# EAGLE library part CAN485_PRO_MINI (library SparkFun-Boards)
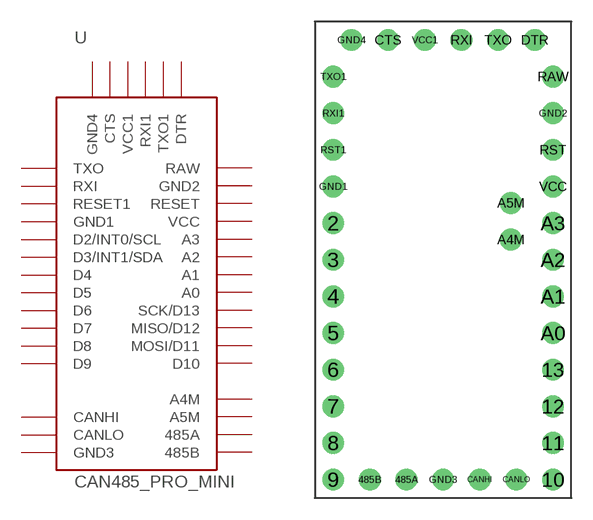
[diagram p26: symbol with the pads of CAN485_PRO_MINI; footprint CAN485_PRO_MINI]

Designator prefix -

## CAN485_PRO_MINIPRO_MINI_COMPATIBLE  [CAN485_PRO_MINI]
2  D2/INT0/SCL
3  D3/INT1/SDA
4  D4
5  D5
6  D6
7  D7
8  D8
9  D9
10  D10
11  MOSI/D11
12  MISO/D12
13  SCK/D13
485A  485A
485B  485B
A0  A0
A1  A1
A2  A2
A3  A3
A4M  A4M
A5M  A5M
CANHI  CANHI
CANLO  CANLO
CTS  CTS
DTR  DTR
GND1  GND1
GND2  GND2
GND3  GND3
GND4  GND4
RAW  RAW
RST  RESET
RST1  RESET1
RXI  RXI
RXI1  RXI1
TXO  TXO
TXO1  TXO1
VCC  VCC
VCC1  VCC1

## Footprint CAN485_PRO_MINI (pad centres in mm)
drill 1: 2 -7.62,3.81; 3 -7.62,1.27; 4 -7.62,-1.27; 5 -7.62,-3.81; 6 -7.62,-6.35; 7 -7.62,-8.89; 8 -7.62,-11.43; 9 -7.62,-13.97; 10 7.62,-13.97; 11 7.62,-11.43; 12 7.62,-8.89; 13 7.62,-6.35; 485A -2.54,-13.97; 485B -5.08,-13.97; A0 7.62,-3.81; A1 7.62,-1.27; A2 7.62,1.27; A3 7.62,3.81; A4M 4.699,2.667; A5M 4.699,5.207; CANHI 2.54,-13.97; CANLO 5.08,-13.97; CTS -3.81,16.51; DTR 6.35,16.51; GND1 -7.62,6.35; GND2 7.62,11.43; GND3 0,-13.97; GND4 -6.35,16.51; RAW 7.62,13.97; RST 7.62,8.89; RST1 -7.62,8.89; RXI 1.27,16.51; RXI1 -7.62,11.43; TXO 3.81,16.51; TXO1 -7.62,13.97; VCC 7.62,6.35; VCC1 -1.27,16.51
